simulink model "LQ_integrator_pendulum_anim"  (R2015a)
settings: Solver=ode45  StartTime=0.0  StopTime=inf  RelTol=1e-3
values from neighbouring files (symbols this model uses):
  g = 9.81    [pendulum_sys_init.m]
  kc = 2    [pendulum_sys_init.m]
  ke = 2    [pendulum_sys_init.m]
  l = 1    [pendulum_sys_init.m]
  M = 10    [pendulum_sys_init.m]
  m = 2    [pendulum_sys_init.m]
  ra = 10    [pendulum_sys_init.m]
  rr = .1    (= 0.1)    [pendulum_sys_init.m]
  T = 0.1    [pendulum_sys_init.m]
undefined symbols (not defined in the file or in its folder): DiscIntNeverNeededParam, float, K, pendolo_sys_diff
libraries: simulink x1, vrlib x1

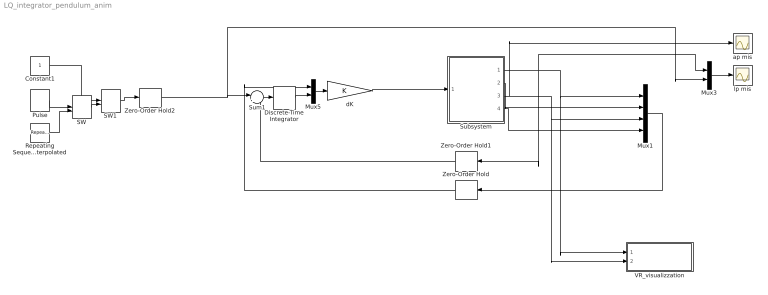
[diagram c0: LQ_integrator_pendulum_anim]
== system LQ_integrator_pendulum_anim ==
  Constant1 : Constant
  Discrete-Time Integrator : DiscreteIntegrator  IntegratorMethod=Accumulation: Forward Euler  InitialConditionSetting=State (most efficient)  SampleTime=T  ICPrevOutput=DiscIntNeverNeededParam  ICPrevScaledInput=DiscIntNeverNeededParam
  Mux1 : Mux
  Mux3 : Mux  Inputs=2
  Mux5 : Mux  Inputs=2
  Pulse : DiscretePulseGenerator  PulseType=Time based  Amplitude=.5  Period=20  PulseWidth=50
  Repeating Sequence Interpolated : simulink/Sources/Repeating Sequence Interpolated  OutValues=[.5 -.5 -.5 .5 .5 -.5 -.5 .5].'  TimeValues=[0 10 15 25 30 40 45 55].'  LookUpMeth=Interpolation-Use End Values  tsamp=0.01  OutMin=[]  OutMax=[]  OutDataTypeStr=float('double')  OutputDataTypeScalingMode=Specify via dialog  OutDataType=float('double')  OutScaling=2^-10
  SW : ManualSwitch
  SW1 : ManualSwitch  CurrentSetting=0
  Subsystem : Subsystem
  Sum1 : Sum  Inputs=|+-
  VR_visualizzation : Subsystem
  Zero-Order Hold : ZeroOrderHold  SampleTime=T
  Zero-Order Hold1 : ZeroOrderHold  SampleTime=T
  Zero-Order Hold2 : ZeroOrderHold  SampleTime=T
  ap mis : Scope
  dK : Gain  Gain=K  Multiplication=Matrix(K*u) (u vector)
  lp mis : Scope
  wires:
  Subsystem/3(ap) -> ap mis/1, Mux1/3, VR_visualizzation/2(ap)
  Subsystem/1(lp) -> Mux3/1, Zero-Order Hold1/1, VR_visualizzation/1(lp), Mux1/1
  Mux3/1 -> lp mis/1
  Constant1/1 -> SW1/1
  Mux1/1 -> Zero-Order Hold/1
  SW1/1 -> Zero-Order Hold2/1
  Sum1/1 -> Discrete-Time Integrator/1
  Discrete-Time Integrator/1 -> Mux5/2
  Mux5/1 -> dK/1
  SW/1 -> SW1/2
  Pulse/1 -> SW/1
  Repeating Sequence Interpolated/1 -> SW/2
  Subsystem/2(lv) -> Mux1/2
  Subsystem/4(av) -> Mux1/4
  dK/1 -> Subsystem/1(voltage)
  Zero-Order Hold/1 -> Mux5/1
  Zero-Order Hold1/1 -> Sum1/2
  Zero-Order Hold2/1 -> Mux3/2, Sum1/1

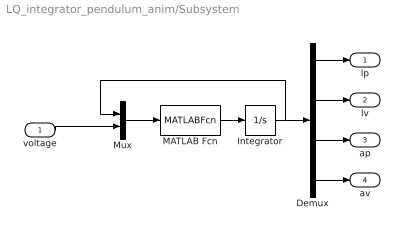
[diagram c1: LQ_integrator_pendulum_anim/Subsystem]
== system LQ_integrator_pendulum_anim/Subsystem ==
  voltage : Inport
  Demux : Demux
  Integrator : Integrator  InitialCondition=[0 0 0.1 0]
  MATLAB Fcn : MATLABFcn  MATLABFcn=pendolo_sys_diff(u,M,m,l,ra,rr,ke,kc,g)
  Mux : Mux  Inputs=2
  lp : Outport
  lv : Outport  Port=2
  ap : Outport  Port=3
  av : Outport  Port=4
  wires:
  MATLAB Fcn/1 -> Integrator/1
  Integrator/1 -> Demux/1, Mux/1
  Demux/4 -> av/1
  Demux/3 -> ap/1
  Demux/2 -> lv/1
  Demux/1 -> lp/1
  Mux/1 -> MATLAB Fcn/1
  voltage/1 -> Mux/2

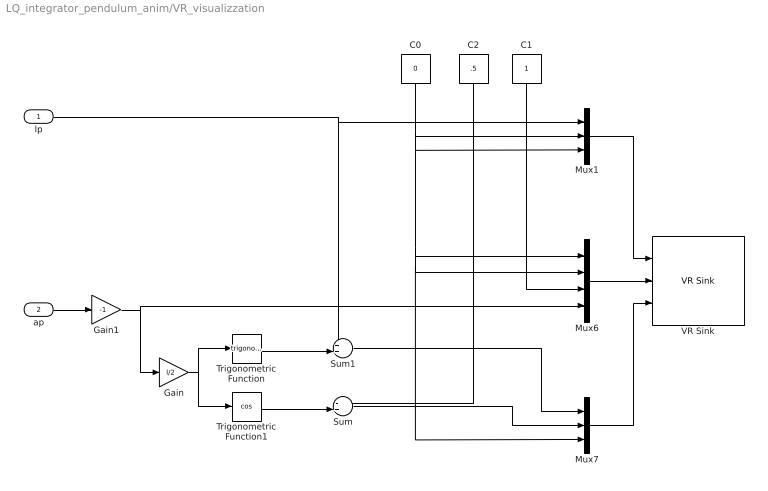
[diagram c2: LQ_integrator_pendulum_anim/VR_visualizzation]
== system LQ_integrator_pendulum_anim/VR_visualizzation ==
  lp : Inport
  ap : Inport  Port=2
  C0 : Constant  Value=0
  C1 : Constant
  C2 : Constant  Value=.5
  Gain : Gain  Gain=l/2
  Gain1 : Gain  Gain=-1
  Mux1 : Mux  Inputs=3
  Mux6 : Mux
  Mux7 : Mux  Inputs=3
  Sum : Sum  Inputs=-+|
  Sum1 : Sum  Inputs=++|
  Trigonometric Function : Trigonometry
  Trigonometric Function1 : Trigonometry  Operator=cos
  VR Sink : vrlib/VR Sink  InstantiateOnLoad=on  SampleTime=0.02  ViewEnable=on  RemoteChange=off  RemoteView=off  FieldsWritten=carrello.translation.3.1.double#asta.rotation.4.1.double#asta.translation.3.1.double  WorldFileName=vrml1.wrl  AutoView=on  VideoDimensions=[]  AllowVariableSize=off  FigureProperties={'Position', 'Name', 'Viewpoint', 'CameraBound', 'CameraDirection', 'CameraPosition', 'CameraUpVector', 'ZoomFactor', 'Antialiasing', 'Headlight', 'Lighting', 'NavPanel', 'Sound', 'StatusBar', 'Stereo3D', 'Stereo3DCameraOffset', 'Stereo3DHIT', 'ToolBar', 'Textures', 'Transparency', 'Triad', 'Wireframe', 'NavZones', 'NavMode', 'NavSpeed', 'CaptureFileFormat', 'CaptureFileName', 'Record2DCompressMet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
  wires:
  Mux1/1 -> VR Sink/1
  Mux6/1 -> VR Sink/2
  Mux7/1 -> VR Sink/3
  lp/1 -> Mux1/1, Sum1/1
  C0/1 -> Mux1/2, Mux1/3, Mux6/1, Mux6/2, Mux7/3
  ap/1 -> Gain1/1
  C1/1 -> Mux6/3
  Trigonometric Function/1 -> Sum1/2
  Trigonometric Function1/1 -> Sum/2
  Sum1/1 -> Mux7/1
  Sum/1 -> Mux7/2
  C2/1 -> Sum/1
  Gain/1 -> Trigonometric Function/1, Trigonometric Function1/1
  Gain1/1 -> Mux6/4, Gain/1
